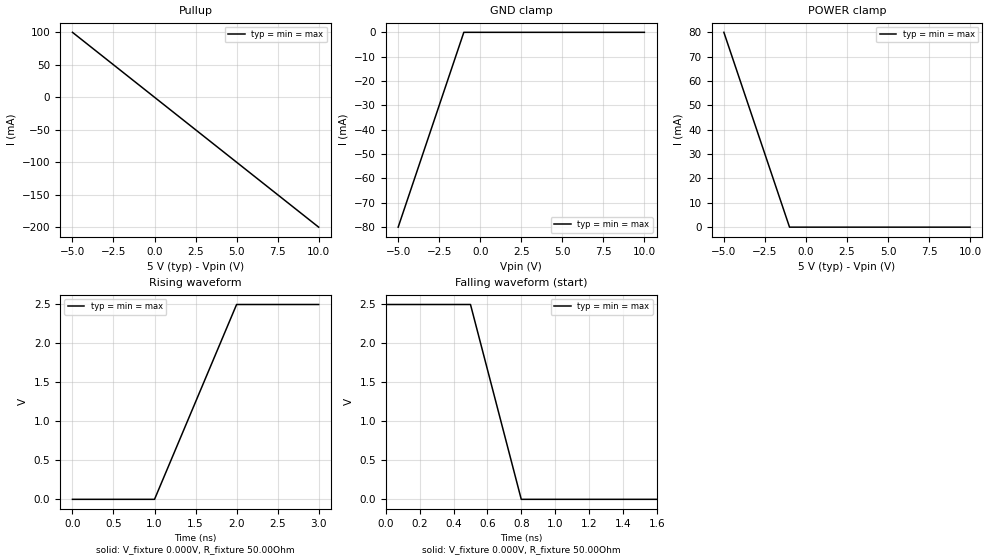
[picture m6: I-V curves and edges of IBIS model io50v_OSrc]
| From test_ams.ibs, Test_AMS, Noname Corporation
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[Model]   io50v_OSrc
Model_type   I/O_open_source
Vinl = 800.000mV
Vinh = 2.000V
Vmeas = 1.400V
Vref = 1.400V
Cref = 0.000F
Rref = 50.000Ohm
|   typ   min   max
C_comp   5.000pF   5.000pF   5.000pF
[Voltage Range]   5.000V   5.000V   5.000V
[Temperature Range]   50.0   100.0   0.0
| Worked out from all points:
|   slope of the pullup table from 0 to 0.75 V, typ, clamps not added: 50 ohm
|   falling waveform, V_fixture 0.000V, R_fixture 50.00Ohm: 20-80 % time 180ps typ, 180ps min, 180ps max; typ from 2.5 V to 0 V
|   rising waveform, V_fixture 0.000V, R_fixture 50.00Ohm: 20-80 % time 600ps typ, 600ps min, 600ps max; typ from 0 V to 2.5 V
[GND Clamp]
|   Voltage   I(typ)   I(min)   I(max)
-5V       -80mA      -80mA      -80mA
-1V       0A         0A         0A
5V        0A         0A         0A
10V       0A         0A         0A
[Pullup]
|   Voltage   I(typ)   I(min)   I(max)
-5V       100mA      100mA      100mA
0V        0A         0A         0A
5V        -100mA     -100mA     -100mA
10V       -200mA     -200mA     -200mA
[POWER Clamp]
|   Voltage   I(typ)   I(min)   I(max)
-5V       80mA       80mA       80mA
-1V       0A         0A         0A
5V        0A         0A         0A
10V       0A         0A         0A
[Ramp]
R_load = 50.00Ohm
|   typ   min   max
dV/dt_r   1.403V/1.248ns   1.116V/1.589ns   1.750V/927.496ps
dV/dt_f   1.513V/1.385ns   1.201V/1.726ns   1.878V/1.020ns
[Falling Waveform]
V_fixture = 0.000V
V_fixture_min = 0.000V
V_fixture_max = 0.000V
R_fixture = 50.00Ohm
|   Time   V(typ)   V(min)   V(max)
0s        2.5V       2.5V       2.5V
500ps     2.5V       2.5V       2.5V
800ps     0V         0V         0V
3ns       0V         0V         0V
[Rising Waveform]
V_fixture = 0.000V
V_fixture_min = 0.000V
V_fixture_max = 0.000V
R_fixture = 50.00Ohm
|   Time   V(typ)   V(min)   V(max)
0s        0V         0V         0V
1ns       0V         0V         0V
2ns       2.5V       2.5V       2.5V
3ns       2.5V       2.5V       2.5V
